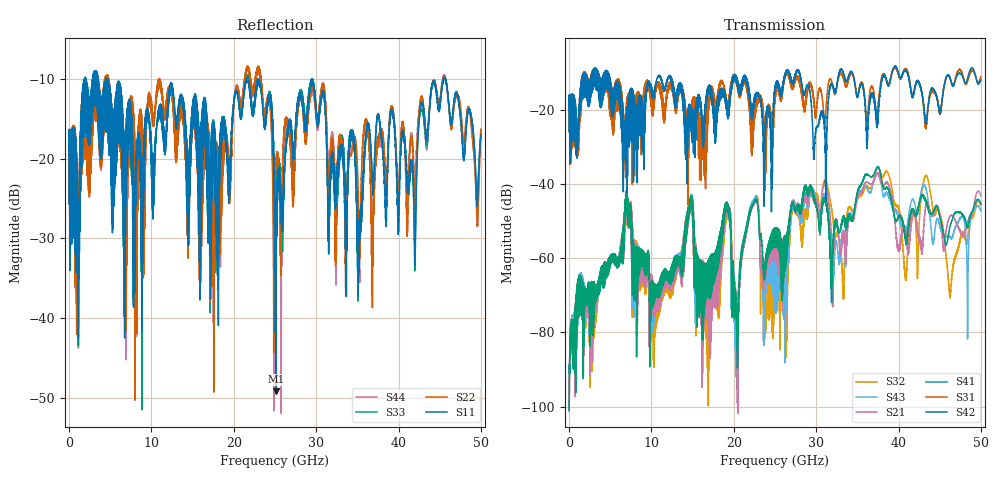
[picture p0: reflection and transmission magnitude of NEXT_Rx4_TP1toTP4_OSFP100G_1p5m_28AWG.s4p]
! Touchstone data
! Created: 27-Feb-2019 by IdEM 12 (12.1.0)
! COMMENTS
!  Created Wed Feb 27 09:43:39 2019
!  64 Port Network Data from SP1.SP block
!  freq  magS1_1  angS1_1  magS1_2  angS1_2  magS1_3  angS1_3  magS1_4  angS1_4
!  magS1_5  angS1_5  magS1_6  angS1_6  magS1_7  angS1_7  magS1_8  angS1_8
!  magS1_9  angS1_9  magS1_10  angS1_10  magS1_11  angS1_11  magS1_12  angS1_12
!  magS1_13  angS1_13  magS1_14  angS1_14  magS1_15  angS1_15  magS1_16  angS1_16
!  magS1_17  angS1_17  magS1_18  angS1_18  magS1_19  angS1_19  magS1_20  angS1_20
!  magS1_21  angS1_21  magS1_22  angS1_22  magS1_23  angS1_23  magS1_24  angS1_24
!  magS1_25  angS1_25  magS1_26  angS1_26  magS1_27  angS1_27  magS1_28  angS1_28
!  magS1_29  angS1_29  magS1_30  angS1_30  magS1_31  angS1_31  magS1_32  angS1_32
!  magS1_33  angS1_33  magS1_34  angS1_34  magS1_35  angS1_35  magS1_36  angS1_36
!  magS1_37  angS1_37  magS1_38  angS1_38  magS1_39  angS1_39  magS1_40  angS1_40
!  magS1_41  angS1_41  magS1_42  angS1_42  magS1_43  angS1_43  magS1_44  angS1_44
!  magS1_45  angS1_45  magS1_46  angS1_46  magS1_47  angS1_47  magS1_48  angS1_48
!  magS1_49  angS1_49  magS1_50  angS1_50  magS1_51  angS1_51  magS1_52  angS1_52
!  magS1_53  angS1_53  magS1_54  angS1_54  magS1_55  angS1_55  magS1_56  angS1_56
!  magS1_57  angS1_57  magS1_58  angS1_58  magS1_59  angS1_59  magS1_60  angS1_60
!  magS1_61  angS1_61  magS1_62  angS1_62  magS1_63  angS1_63  magS1_64  angS1_64
!  magS2_1  angS2_1  magS2_2  angS2_2  magS2_3  angS2_3  magS2_4  angS2_4
!  magS2_5  angS2_5  magS2_6  angS2_6  magS2_7  angS2_7  magS2_8  angS2_8
!  magS2_9  angS2_9  magS2_10  angS2_10  magS2_11  angS2_11  magS2_12  angS2_12
!  magS2_13  angS2_13  magS2_14  angS2_14  magS2_15  angS2_15  magS2_16  angS2_16
!  magS2_17  angS2_17  magS2_18  angS2_18  magS2_19  angS2_19  magS2_20  angS2_20
!  magS2_21  angS2_21  magS2_22  angS2_22  magS2_23  angS2_23  magS2_24  angS2_24
!  magS2_25  angS2_25  magS2_26  angS2_26  magS2_27  angS2_27  magS2_28  angS2_28
!  magS2_29  angS2_29  magS2_30  angS2_30  magS2_31  angS2_31  magS2_32  angS2_32
!  magS2_33  angS2_33  magS2_34  angS2_34  magS2_35  angS2_35  magS2_36  angS2_36
!  magS2_37  angS2_37  magS2_38  angS2_38  magS2_39  angS2_39  magS2_40  angS2_40
!  magS2_41  angS2_41  magS2_42  angS2_42  magS2_43  angS2_43  magS2_44  angS2_44
!  magS2_45  angS2_45  magS2_46  angS2_46  magS2_47  angS2_47  magS2_48  angS2_48
!  magS2_49  angS2_49  magS2_50  angS2_50  magS2_51  angS2_51  magS2_52  angS2_52
!  magS2_53  angS2_53  magS2_54  angS2_54  magS2_55  angS2_55  magS2_56  angS2_56
!  magS2_57  angS2_57  magS2_58  angS2_58  magS2_59  angS2_59  magS2_60  angS2_60
!  magS2_61  angS2_61  magS2_62  angS2_62  magS2_63  angS2_63  magS2_64  angS2_64
!  magS3_1  angS3_1  magS3_2  angS3_2  magS3_3  angS3_3  magS3_4  angS3_4
!  magS3_5  angS3_5  magS3_6  angS3_6  magS3_7  angS3_7  magS3_8  angS3_8
!  magS3_9  angS3_9  magS3_10  angS3_10  magS3_11  angS3_11  magS3_12  angS3_12
!  magS3_13  angS3_13  magS3_14  angS3_14  magS3_15  angS3_15  magS3_16  angS3_16
!  magS3_17  angS3_17  magS3_18  angS3_18  magS3_19  angS3_19  magS3_20  angS3_20
!  magS3_21  angS3_21  magS3_22  angS3_22  magS3_23  angS3_23  magS3_24  angS3_24
!  magS3_25  angS3_25  magS3_26  angS3_26  magS3_27  angS3_27  magS3_28  angS3_28
!  magS3_29  angS3_29  magS3_30  angS3_30  magS3_31  angS3_31  magS3_32  angS3_32
!  magS3_33  angS3_33  magS3_34  angS3_34  magS3_35  angS3_35  magS3_36  angS3_36
!  magS3_37  angS3_37  magS3_38  angS3_38  magS3_39  angS3_39  magS3_40  angS3_40
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# Hz S MA R 50
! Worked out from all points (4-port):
!   5000 points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, 10 MHz to 50 GHz, reference 50 ohm
!   strongest paths, dB at 10 MHz, 12.51 GHz, 25.01 GHz, 37.51 GHz, 50 GHz:
!     S42: -19.6, -12.6, -13.6, -21.6, -11.9
!     S31: -19.6, -14.0, -15.9, -19.1, -11.0
!     S41: -101.0, -66.0, -52.7, -35.3, -45.3
!     S21: -101.0, -68.0, -55.1, -37.1, -43.1
!     S43: -101.3, -67.5, -56.9, -35.4, -47.3
!     S32: -100.7, -69.9, -60.7, -35.6, -45.6
!   lowest |S11| = -49.2 dB at 25.11 GHz (marker M1), VSWR 1.01, Z = 50.3 + j0.113 ohm
!   |S11| at or under -10 dB: 4.66 GHz to 21.51 GHz (16.85 GHz wide, 129 % of centre); 22.94 GHz to 45.47 GHz (22.53 GHz wide, 65.9 % of centre); 45.68 GHz to end of sweep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
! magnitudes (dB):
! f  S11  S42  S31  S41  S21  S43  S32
! 10 MHz  -19.2  -19.6  -19.6  -101.0  -101.0  -101.3  -100.7
! 7.07 GHz  -14.4  -19.3  -17.3  -43.7  -44.7  -44.5  -45.3
! 10.01 GHz  -19.8  -14.2  -16.6  -73.6  -72.4  -80.0  -78.1
! 14.79 GHz  -19.2  -21.4  -19.8  -43.3  -43.6  -43.0  -43.4
! 20.32 GHz  -11.6  -12.4  -12.9  -72.4  -73.1  -86.5  -92.0
! 25.11 GHz  -49.2  -12.7  -14.8  -52.8  -55.4  -56.9  -60.8
! 50 GHz  -17.1  -11.9  -11.0  -45.3  -43.1  -47.3  -45.6
